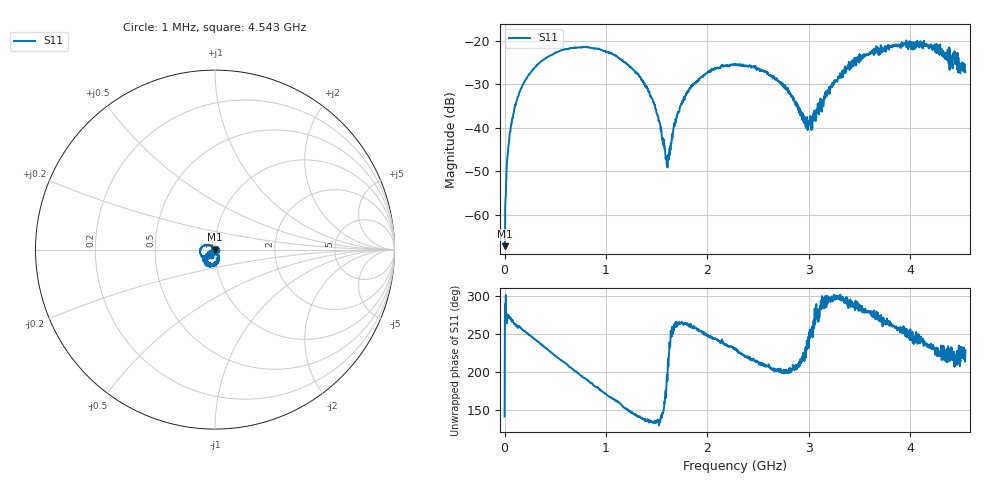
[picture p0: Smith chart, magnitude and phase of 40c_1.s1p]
# HZ S RI R 50
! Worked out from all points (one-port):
!   1515 points, 1 MHz to 4.543 GHz, reference 50 ohm
!   lowest |S11| = -67.3 dB at 4 MHz (marker M1), VSWR 1.00, Z = 50 - j0.0431 ohm
!   |S11| at or under -10 dB: start of sweep to end of sweep
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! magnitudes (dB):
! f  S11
! 1 MHz  -66.5
! 4 MHz  -67.3
! 28 MHz  -46.8
! 46 MHz  -42.7
! 85 MHz  -37.0
! 136 MHz  -32.7
! 313 MHz  -25.7
! 571 MHz  -22.0
! 913 MHz  -21.8
! 1.138 GHz  -24.1
! 1.411 GHz  -31.2
! 1.513 GHz  -37.3
! 1.6 GHz  -48.5
! 1.621 GHz  -47.3
! 1.705 GHz  -36.9
! 1.81 GHz  -31.6
! 1.936 GHz  -28.3
! 2.272 GHz  -25.4
! 2.572 GHz  -27.1
! 2.842 GHz  -33.0
! 2.956 GHz  -37.9
! 3.013 GHz  -39.4
! 3.232 GHz  -29.8
! 3.409 GHz  -26.1
! 3.658 GHz  -22.3
! 3.976 GHz  -21.7
! 4.291 GHz  -22.2
! 4.543 GHz  -27.2
